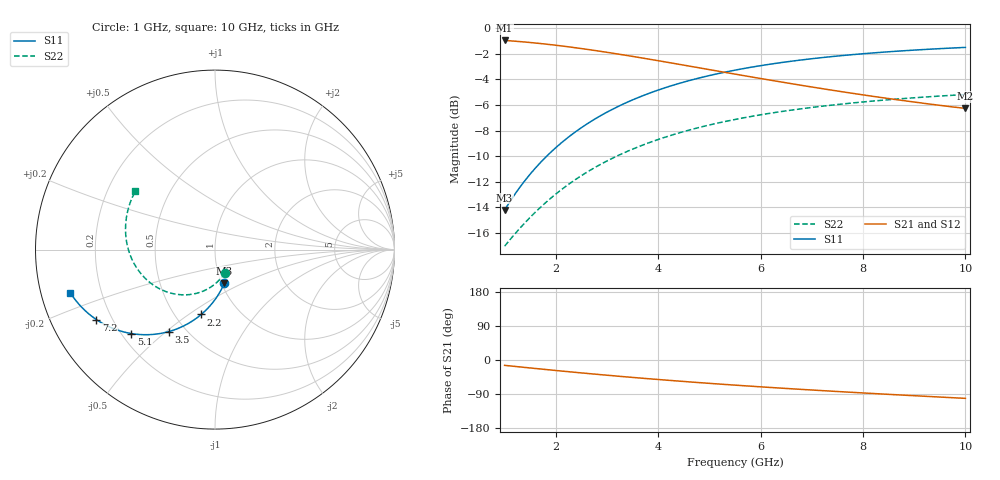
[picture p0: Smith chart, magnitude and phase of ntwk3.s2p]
! Created Thu Nov 11 11:19:04 2010
# ghz S ri R 50
! 2 Port Network Data from SP1.SP block
! freq  reS11  imS11  reS21  imS21  reS12  imS12  reS22  imS22
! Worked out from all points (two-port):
!   91 points, 1 GHz to 10 GHz, reference 50 ohm
!   highest |S21| = -0.96 dB at 1 GHz (marker M1); lowest = -6.3 dB at 10 GHz (marker M2)
!   |S21| within 3 dB of the highest: start of sweep to 6.043 GHz
!   lowest |S11| = -14.2 dB at 1 GHz (marker M3), VSWR 1.48, Z = 51.5 - j20.1 ohm
!   |S11| at or under -10 dB: start of sweep to 1.821 GHz
!   |S22| runs from -17.0 to -5.2 dB; largest |S21 - S12| = 0
!   S11 on the Smith chart (normalised r, x): 1 GHz: 1.03, -0.40; 2.2 GHz: 0.67, -0.56; 3.5 GHz: 0.40, -0.51; 5.1 GHz: 0.24, -0.40; 7.2 GHz: 0.14, -0.27; 10 GHz: 0.09, -0.15
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1  0.052 -0.1879  0.8681 -0.2188  0.8681 -0.2188  0.0535 -0.1304
1.1  0.0441 -0.2051  0.8598 -0.239  0.8598 -0.239  0.046 -0.1417
1.3  0.0265 -0.2382  0.8413 -0.2781  0.8413 -0.2781  0.0292 -0.1631
1.6  -0.00398 -0.2841  0.8091 -0.3329  0.8091 -0.3329  0.000248 -0.1912
1.9  -0.0387 -0.3252  0.7724 -0.3827  0.7724 -0.3827  -0.0324 -0.2143
2.2  -0.0767 -0.3611  0.7323 -0.4272  0.7323 -0.4272  -0.0678 -0.2319
2.5  -0.117 -0.3918  0.6896 -0.4661  0.6896 -0.4661  -0.105 -0.244
3  -0.1871 -0.4312  0.615 -0.5189  0.615 -0.5189  -0.1683 -0.2521
3.5  -0.2581 -0.4569  0.5393 -0.5575  0.5393 -0.5575  -0.2304 -0.2461
4  -0.3273 -0.4706  0.465 -0.5836  0.465 -0.5836  -0.2885 -0.2279
4.5  -0.3929 -0.4742  0.394 -0.5991  0.394 -0.5991  -0.3406 -0.1995
5.1  -0.4656 -0.4677  0.3147 -0.6064  0.3147 -0.6064  -0.3938 -0.155
5.5  -0.5098 -0.4582  0.2658 -0.6059  0.2658 -0.6059  -0.4232 -0.1206
5.8  -0.5408 -0.449  0.2312 -0.6032  0.2312 -0.6032  -0.4419 -0.0929
6.2  -0.5792 -0.4343  0.188 -0.5972  0.188 -0.5972  -0.4626 -0.0541
6.6  -0.6143 -0.4176  0.1478 -0.5889  0.1478 -0.5889  -0.4784 -0.0138
7  -0.6463 -0.3992  0.1106 -0.5788  0.1106 -0.5788  -0.4895 0.0274
7.2  -0.6612 -0.3895  0.0931 -0.5732  0.0931 -0.5732  -0.4934 0.0482
7.8  -0.7016 -0.3592  0.0444 -0.5547  0.0444 -0.5547  -0.4984 0.1106
8.5  -0.7417 -0.322  -0.00592 -0.5311  -0.00592 -0.5311  -0.4928 0.1825
9.2  -0.7749 -0.2842  -0.0501 -0.5061  -0.0501 -0.5061  -0.4758 0.2517
10  -0.8058 -0.2409  -0.0945 -0.4767  -0.0945 -0.4767  -0.4436 0.3261
